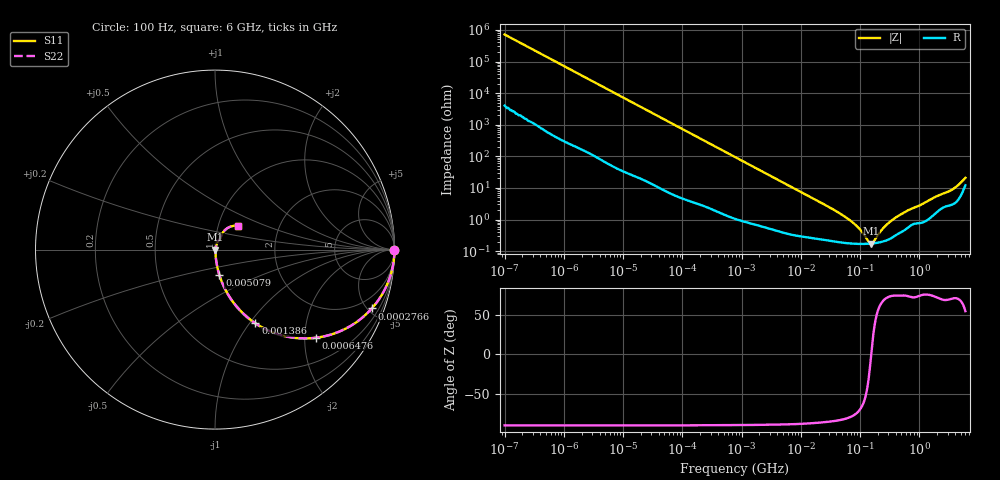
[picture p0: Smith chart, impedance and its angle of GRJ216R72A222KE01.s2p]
!Murata Part Number: GRJ216R72A222KE01
!These Parameters are Measured in Series Mode Connection
!Data Generated on Jun 19, 2026
!  o--ll--o
!Port1  Port2
!  o------o
!Operation Temp=25[degC], DC Bias Voltage=0[V]
!Freq. Start=100[Hz] Stop=6[GHz] 401[Steps]
# Hz S RI R 50
!Freq.(Hz) S11(Real) S11(Imag) S21(Real) S21(Imag) S12(Real) S12(Imag) S22(Real) S22(Imag)
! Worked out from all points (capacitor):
!   401 points, 100 Hz to 6 GHz, reference 50 ohm
!   read as one part in series: C = 2.22 nF near 109 Hz
!   lowest |Z| = 174 mohm at 152.6 MHz (marker M1)
!   series resonance near 154.4 MHz, so ESL is about 480 pH
!   S11 on the Smith chart (normalised r, x): 100 Hz: open; 276.6 kHz: 1.05, -5.31; 647.6 kHz: 1.02, -2.28; 1.386 MHz: 1.02, -1.07; 5.079 MHz: 1.01, -0.29; 6 GHz: 1.24, +0.34
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100  1 -0.00014  8e-07 0.00014  8e-07 0.00014  1 -0.00014
2008  1 -0.00278  2.04e-05 0.00278  2.04e-05 0.00278  1 -0.00278
40335  0.9966 -0.0551  0.00336 0.0551  0.00336 0.0551  0.9966 -0.0551
112960  0.9757 -0.1506  0.0243 0.1506  0.0243 0.1506  0.9757 -0.1506
276587  0.8735 -0.328  0.1265 0.328  0.1265 0.328  0.8735 -0.328
413847  0.7576 -0.4238  0.2424 0.4238  0.2424 0.4238  0.7576 -0.4238
647581  0.5639 -0.4907  0.4361 0.4907  0.4361 0.4907  0.5639 -0.4907
774597  0.4761 -0.4939  0.5239 0.4939  0.5239 0.4939  0.4761 -0.4939
1386327  0.2251 -0.4106  0.7749 0.4106  0.7749 0.4106  0.2251 -0.4106
2481164  0.0867 -0.2722  0.9133 0.2722  0.9133 0.2722  0.0867 -0.2722
5079039  0.0248 -0.1431  0.9752 0.1431  0.9752 0.1431  0.0248 -0.1431
1.555665e7  0.00489 -0.0478  0.9951 0.0478  0.9951 0.0478  0.00489 -0.0478
6.817316e7  0.00183 -0.00917  0.9982 0.00917  0.9982 0.00917  0.00183 -0.00917
9.326766e7  0.00172 -0.00531  0.9983 0.00531  0.9983 0.00531  0.00172 -0.00531
1.395531e8  0.00172 -0.00103  0.9983 0.00103  0.9983 0.00103  0.00172 -0.00103
1.526266e8  0.00174 -0.000117  0.9983 0.000117  0.9983 0.000117  0.00174 -0.000117
1.669249e8  0.00177 0.000792  0.9982 -0.000792  0.9982 -0.000792  0.00177 0.000792
2.283698e8  0.00197 0.00408  0.998 -0.00408  0.998 -0.00408  0.00197 0.00408
3.124326e8  0.00245 0.0078  0.9975 -0.0078  0.9975 -0.0078  0.00245 0.0078
6.395615e8  0.00582 0.0184  0.9942 -0.0184  0.9942 -0.0184  0.00582 0.0184
3.505958e9  0.0344 0.0762  0.9656 -0.0762  0.9656 -0.0762  0.0344 0.0762
6e9  0.1286 0.1326  0.8714 -0.1326  0.8714 -0.1326  0.1286 0.1326
